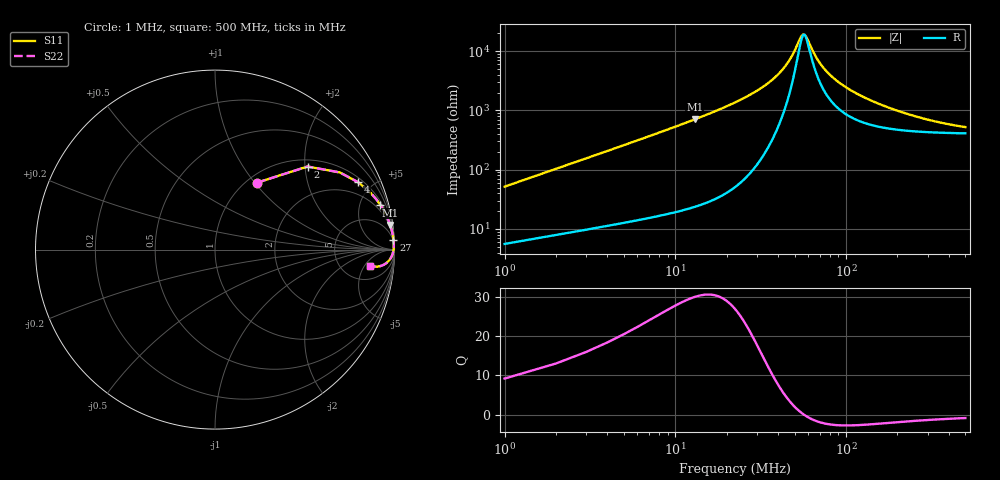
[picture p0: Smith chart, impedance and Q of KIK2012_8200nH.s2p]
!version-2
!date-01.2022
!Series
# MHz S RI R 50
!Freq ReS11 ImS11 ReS21 ImS21 ReS12 ImS12 ReS22 ImS22
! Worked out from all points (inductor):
!   500 points, 1 MHz to 500 MHz, reference 50 ohm
!   read as one part in series: L = 8.2 uH near 3 MHz
!   highest Q = 29.9 at 13 MHz (marker M1), where L = 8.66 uH
!   self-resonance near 56 MHz
!   S11 on the Smith chart (normalised r, x): 1 MHz: 1.11, +1.03; 2 MHz: 1.16, +2.06; 4 MHz: 1.23, +4.14; 7 MHz: 1.31, +7.33; 27 MHz: 3, +36; 500 MHz: 9, -7
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1  0.2352 0.3733  0.7648 -0.3733  0.7648 -0.3733  0.2352 0.3733
2  0.5159 0.4628  0.4841 -0.4628  0.4841 -0.4628  0.5159 0.4628
4  0.7987 0.3747  0.2013 -0.3747  0.2013 -0.3747  0.7987 0.3747
5  0.8593 0.3241  0.1407 -0.3241  0.1407 -0.3241  0.8593 0.3241
7  0.9218 0.2484  0.0782 -0.2484  0.0782 -0.2484  0.9218 0.2484
13  0.976 0.1372  0.024 -0.1372  0.024 -0.1372  0.976 0.1372
27  0.9944 0.055  0.00561 -0.055  0.00561 -0.055  0.9944 0.055
42  0.9962 0.0207  0.00379 -0.0207  0.00379 -0.0207  0.9962 0.0207
47  0.996 0.0129  0.00405 -0.0129  0.00405 -0.0129  0.996 0.0129
54  0.9952 0.00355  0.00479 -0.00355  0.00479 -0.00355  0.9952 0.00355
56  0.9949 0.00114  0.00506 -0.00114  0.00506 -0.00114  0.9949 0.00114
59  0.9945 -0.00231  0.00552 0.00231  0.00552 0.00231  0.9945 -0.00231
65  0.9934 -0.00867  0.00657 0.00867  0.00657 0.00867  0.9934 -0.00867
71  0.9922 -0.0145  0.00779 0.0145  0.00779 0.0145  0.9922 -0.0145
85  0.9888 -0.0263  0.0112 0.0263  0.0112 0.0263  0.9888 -0.0263
99  0.9848 -0.0363  0.0152 0.0363  0.0152 0.0363  0.9848 -0.0363
117  0.979 -0.0474  0.021 0.0474  0.021 0.0474  0.979 -0.0474
168  0.96 -0.0705  0.04 0.0705  0.04 0.0705  0.96 -0.0705
251  0.9274 -0.0898  0.0726 0.0898  0.0726 0.0898  0.9274 -0.0898
334  0.8992 -0.0951  0.1008 0.0951  0.1008 0.0951  0.8992 -0.0951
417  0.8773 -0.0934  0.1227 0.0934  0.1227 0.0934  0.8773 -0.0934
500  0.8609 -0.0886  0.1391 0.0886  0.1391 0.0886  0.8609 -0.0886
